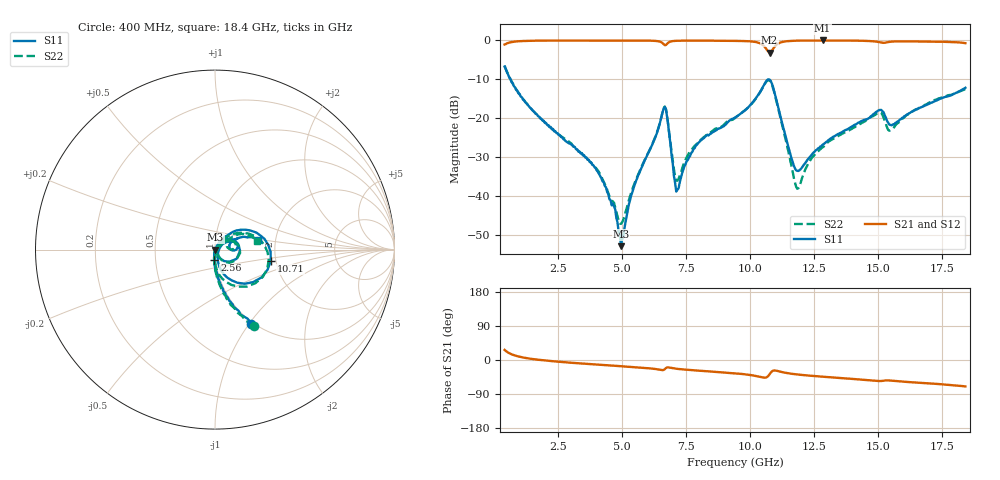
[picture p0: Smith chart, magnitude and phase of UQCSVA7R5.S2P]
!  Part Number  UQCSVA7R5  Mounting Orientation: Horizontal
!  Description: Ultra Low ESR Microwave capacitors
!  Application: Coupling, Bypass, Tuning, DC Block
!  Filters, Matching
# GHZ S DB R 50
! Freq  |S11|  S11 Ph  |S21|  S21 Ph  |S12|  S12 Ph  |S22|  S22 Ph
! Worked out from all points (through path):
!   401 points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, 400 MHz to 18.4 GHz, reference 50 ohm
!   highest |S21| = 0.00 dB at 12.82 GHz (marker M1); lowest = -3.1 dB at 10.75 GHz (marker M2)
!   group delay of S21, straight-line fit = 11.3 ps
!   lowest |S11| = -52.9 dB at 4.945 GHz (marker M3), VSWR 1.00, Z = 50.2 - j0.0878 ohm
!   |S11| at or under -10 dB: 628.7 MHz to 10.7 GHz (10.07 GHz wide, 178 % of centre); 10.71 GHz to end of sweep
!   |S22| runs from -47.2 to -6.5 dB; largest |S21 - S12| = 0.019
!   S11 on the Smith chart (normalised r, x): 400 MHz: 0.97, -1.03; 2.56 GHz: 0.99, -0.12; 10.71 GHz: 1.88, -0.26; 18.4 GHz: 1.62, +0.19
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0.4  -6.72 -63.9  -1.05 26.6  -0.90 26.0  -6.46 -62.9
1.12  -15.23 -83.3  -0.14 6.7  -0.12 5.7  -15.06 -84.1
2.56  -24.42 -93.4  -0.02 -4.8  -0.06 -5.1  -24.38 -94.0
3.415  -28.98 -95.8  -0.02 -9.3  -0.05 -9.4  -29.06 -96.3
4.27  -36.42 -99.0  -0.01 -13.2  -0.04 -13.3  -36.34 -97.3
4.945  -52.92 -22.8  -0.01 -16.3  -0.03 -16.4  -47.18 -22.1
5.44  -37.91 59.2  -0.02 -18.7  -0.03 -18.7  -37.36 44.6
6.43  -22.13 47.2  -0.23 -25.2  -0.22 -25.3  -21.96 40.7
6.7  -17.68 -23.2  -1.18 -21.4  -1.19 -21.7  -17.60 -27.0
7.15  -38.38 2.0  -0.08 -23.4  -0.11 -23.4  -36.06 -5.1
7.96  -26.38 58.3  -0.04 -28.0  -0.06 -28.0  -26.17 47.0
9.4  -19.84 49.2  -0.11 -35.2  -0.13 -35.2  -19.96 46.2
10.39  -13.12 29.1  -0.78 -44.7  -0.79 -44.6  -13.23 22.6
10.705  -9.98 -11.4  -2.91 -41.8  -2.91 -41.6  -10.17 -19.8
10.75  -10.07 -21.0  -3.10 -37.7  -3.07 -37.6  -10.25 -29.6
11.11  -17.82 -72.6  -0.72 -29.8  -0.72 -29.8  -18.16 -83.3
11.785  -33.40 -30.6  -0.06 -37.8  -0.07 -37.8  -37.54 -44.2
12.415  -29.27 28.0  -0.02 -41.9  -0.01 -41.9  -30.07 34.3
12.82  -26.86 34.4  0.00 -44.1  -0.01 -44.0  -27.50 39.5
15.025  -17.94 14.4  -0.41 -55.5  -0.42 -55.1  -18.60 17.4
15.43  -21.65 4.2  -0.36 -54.0  -0.35 -53.8  -23.22 14.5
18.4  -12.18 12.9  -0.70 -69.7  -0.69 -69.9  -12.50 12.2
